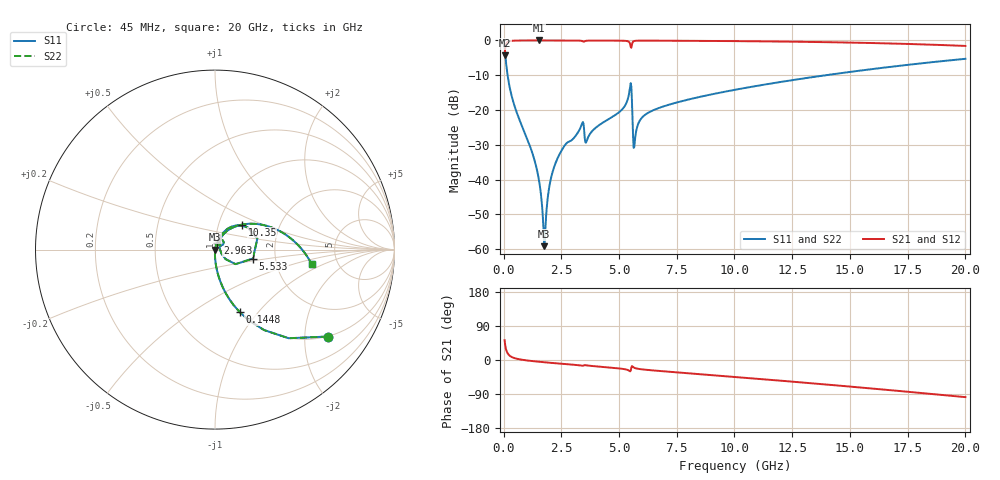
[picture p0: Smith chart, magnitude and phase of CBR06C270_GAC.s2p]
! S-parameter model data by Modelithics Inc.  support@modelithics.com 813-866-6335  Tampa FL USA
! S-Parameter data specifications:
! Substrate: 20-mil Rogers 4350B, substrate thickness, H=0.508mm, Dielectric constant, Er=3.75
! PCB Mounting Pad Footprint: Pad width, PadW=0.85mm , Pad length, PadL=0.64mm , Pad gap, PadG (edge-to-edge)=0.62mm , Reference planes=1.9mm apart
#  GHz  S  MA  R 50
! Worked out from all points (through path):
!   801 points, 45 MHz to 20 GHz, reference 50 ohm
!   highest |S21| = -0.01 dB at 1.542 GHz (marker M1); lowest = -4.3 dB at 45 MHz (marker M2)
!   group delay of S21, straight-line fit = 14.1 ps
!   lowest |S11| = -59.1 dB at 1.766 GHz (marker M3), VSWR 1.00, Z = 50.1 - j0.0242 ohm
!   |S11| at or under -10 dB: 174.6 MHz to 13.96 GHz (13.78 GHz wide, 195 % of centre)
!   |S22| runs from -59.1 to -2.0 dB; largest |S21 - S12| = 0
!   S11 on the Smith chart (normalised r, x): 45 MHz: 0.99, -2.60; 144.8 MHz: 0.99, -0.80; 2.963 GHz: 1.02, +0.07; 5.533 GHz: 1.53, -0.16; 10.35 GHz: 1.29, +0.37; 20 GHz: 3.20, -0.73
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0.045  0.7935 -37.6  0.6084 52.4  0.6084 52.4  0.7935 -37.6
0.144775  0.3736 -68.5  0.9272 21.4  0.9272 21.4  0.3736 -68.5
0.518931  0.103 -85.5  0.994 4.2  0.994 4.2  0.103 -85.5
1.2423  0.02429 -90.7  0.9987 -2.8  0.9987 -2.8  0.02429 -90.7
1.541625  0.009431 -88.5  0.9989 -4.7  0.9989 -4.7  0.009431 -88.5
1.766119  0.001104 -12.6  0.9988 -6.0  0.9988 -6.0  0.001104 -12.6
1.990612  0.00827 74.4  0.9987 -7.2  0.9987 -7.2  0.00827 74.4
2.190163  0.01518 76.6  0.9984 -8.3  0.9984 -8.3  0.01518 76.6
2.963419  0.03716 69.7  0.9939 -12.2  0.9939 -12.2  0.03716 69.7
3.387462  0.06237 62.1  0.9841 -15.0  0.9841 -15.0  0.06237 62.1
3.611956  0.03694 62.9  0.991 -14.3  0.991 -14.3  0.03694 62.9
5.133525  0.1018 64.5  0.9905 -23.2  0.9905 -23.2  0.1018 64.5
5.43285  0.1714 50.7  0.9521 -28.0  0.9521 -28.0  0.1714 50.7
5.532625  0.2171 -13.2  0.7839 -20.2  0.7839 -20.2  0.2171 -13.2
5.707231  0.04181 52.5  0.9874 -21.6  0.9874 -21.6  0.04181 52.5
5.981612  0.07682 62.7  0.9931 -24.6  0.9931 -24.6  0.07682 62.7
6.704981  0.1062 60.0  0.9916 -28.7  0.9916 -28.7  0.1062 60.0
10.0225  0.1953 44.4  0.9775 -44.8  0.9775 -44.8  0.1953 44.4
10.34677  0.2044 42.9  0.9756 -46.4  0.9756 -46.4  0.2044 42.9
13.36496  0.2965 27.8  0.9511 -61.5  0.9511 -61.5  0.2965 27.8
16.68248  0.4143 10.2  0.9054 -79.2  0.9054 -79.2  0.4143 10.2
20  0.5442 -8.5  0.8333 -98.0  0.8333 -98.0  0.5442 -8.5
